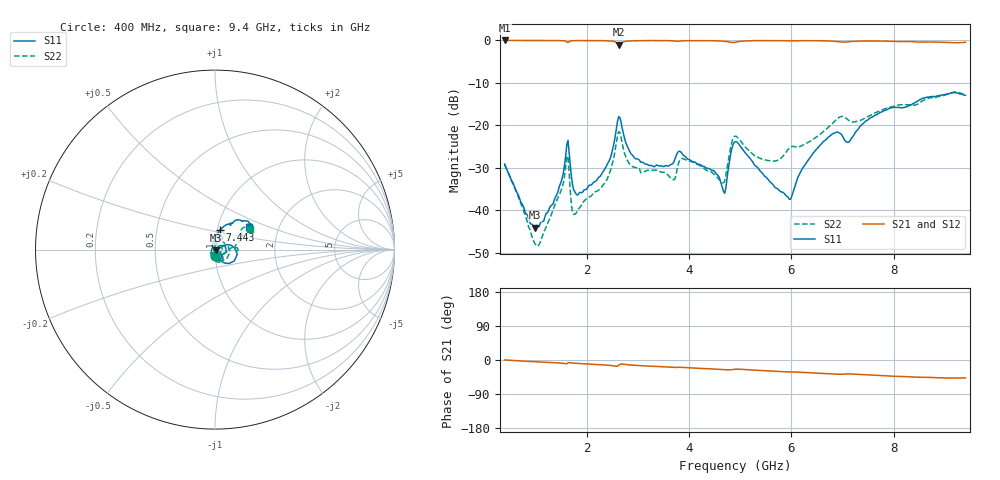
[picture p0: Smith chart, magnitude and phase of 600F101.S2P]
!  American Technical Ceramics  Date:  11/23/05
!  One Norden Lane
!  Huntington Station,  NY.  11746-2102
!  Tel:  (631) 622-4700  Fax:  (631) 622-4748
!  Part Number  600F101  Mounting Orientation: Horizontal
!  Description: Ultra Low ESR Microwave capacitors
!  Application: Coupling, Bypass, Tuning, DC Block
!  Filters, Matching
# GHZ S DB R 50
! Freq  |S11|  S11 Ph  |S21|  S21 Ph  |S12|  S12 Ph  |S22|  S22 Ph
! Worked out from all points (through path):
!   401 points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, 400 MHz to 9.4 GHz, reference 50 ohm
!   highest |S21| = 0.00 dB at 400 MHz (marker M1); lowest = -1.0 dB at 2.628 GHz (marker M2)
!   group delay of S21, straight-line fit = 14.9 ps
!   lowest |S11| = -44.1 dB at 985 MHz (marker M3), VSWR 1.01, Z = 50.6 - j0.291 ohm
!   |S11| at or under -10 dB: start of sweep to end of sweep
!   |S22| runs from -48.4 to -12.1 dB; largest |S21 - S12| = 0.0048
!   S11 on the Smith chart (normalised r, x): 400 MHz: 1.00, -0.07; 7.443 GHz: 1.03, +0.23; 9.4 GHz: 1.41, +0.37
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0.4  -29.08 -86.3  0.00 0.2  -0.02 0.1  -29.24 -89.3
0.985  -44.09 -27.4  0.00 -4.5  -0.02 -4.5  -47.70 -146.6
1.39  -36.93 35.7  -0.01 -7.2  -0.03 -7.3  -38.46 117.6
1.615  -24.46 20.5  -0.35 -9.7  -0.36 -9.7  -27.52 41.4
1.75  -35.20 -30.9  -0.05 -8.3  -0.05 -8.3  -40.93 -154.2
1.908  -35.85 -0.8  -0.03 -9.7  -0.03 -9.7  -38.63 153.6
2.403  -29.20 21.2  -0.09 -13.6  -0.09 -13.6  -32.66 112.8
2.628  -17.95 -12.2  -0.99 -14.3  -1.00 -14.2  -21.45 -8.1
2.92  -27.37 -63.0  -0.08 -13.9  -0.09 -13.9  -29.77 -135.5
3.415  -29.57 -67.1  -0.02 -17.5  -0.03 -17.4  -30.76 -130.5
3.685  -28.98 -59.8  -0.09 -19.4  -0.09 -19.3  -32.74 -116.5
3.82  -26.07 -72.8  -0.14 -19.3  -0.14 -19.3  -28.15 -102.1
4.675  -35.53 -74.7  -0.18 -25.4  -0.18 -25.4  -33.52 -65.2
4.9  -23.84 -68.7  -0.44 -24.4  -0.42 -24.4  -22.52 -64.0
5.53  -32.48 -149.8  -0.03 -28.6  -0.01 -28.6  -28.23 -62.5
5.958  -37.34 130.4  -0.11 -31.4  -0.09 -31.5  -25.37 -24.8
6.408  -26.85 101.1  -0.05 -33.9  -0.05 -34.1  -23.43 -5.4
6.948  -21.84 60.3  -0.33 -37.6  -0.34 -37.5  -18.01 3.3
7.105  -24.02 66.2  -0.32 -36.8  -0.32 -36.6  -18.65 -3.4
7.443  -19.07 76.0  -0.13 -39.0  -0.11 -38.9  -18.21 14.1
7.915  -15.97 63.1  -0.19 -42.4  -0.16 -42.5  -15.78 21.6
9.4  -12.91 33.8  -0.42 -47.2  -0.41 -47.5  -12.87 30.9
